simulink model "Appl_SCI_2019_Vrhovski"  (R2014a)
settings: Solver=ode45  StartTime=0.0  StopTime=1000  MaxStep=0.01  RelTol=1e-3
undefined symbols (not defined in the file): deg, H, kg, m, M, mm, N, rad, s, X, Y, Z
libraries: sm_lib x389, nesl_utility x69, simulink x7
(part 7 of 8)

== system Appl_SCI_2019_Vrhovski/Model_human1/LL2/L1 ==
  Mux : Mux  Inputs=3
  Pos X Converter : nesl_utility/PS-Simulink Converter  PhysicalDomain=network_engine_domain  SubClassName=ps_output  LeftPortType=input  RightPortType=output  PseudoPeriodic=off  Frequencies=[]  Unit=mm  AffineConversion=off
  Pos Y Converter : nesl_utility/PS-Simulink Converter  PhysicalDomain=network_engine_domain  SubClassName=ps_output  LeftPortType=input  RightPortType=output  PseudoPeriodic=off  Frequencies=[]  Unit=mm  AffineConversion=off
  Pos Z Converter2 : nesl_utility/PS-Simulink Converter  PhysicalDomain=network_engine_domain  SubClassName=ps_output  LeftPortType=input  RightPortType=output  PseudoPeriodic=off  Frequencies=[]  Unit=mm  AffineConversion=off
  Transform Sensor : sm_lib/Frames and Transforms/Transform Sensor  MeasurementFrame=World  SenseAngle=off  SenseAxis=off  SenseAngle1=off  SenseAngle2=off  SenseAngle3=off  SenseQ=off  SenseR=off  SenseOmegaX=off  SenseOmegaY=off  SenseOmegaZ=off  SenseOmega1=off  SenseOmega2=off  SenseOmega3=off  SenseQDot=off  SenseRDot=off  SenseAlphaX=off  SenseAlphaY=off  SenseAlphaZ=off  SenseAlpha1=off  SenseAlpha2=off  SenseAlpha3=off  SenseQDDot=off  SenseRDDot=off  SenseX=on  SenseY=on  SenseZ=on  SenseRad=on  SenseAzim=off  SenseDist=off  SenseInc=off  SenseXDot=off  SenseYDot=off  SenseZDot=off  SenseRadDot=off  SenseAzimDot=off  SenseDistDot=off  SenseIncDot=off  SenseXDDot=off  SenseYDDot=off  SenseZDDot=off  SenseRadDDot=off  SenseAzimDDot=off  SenseDistDDot=off  SenseIncDDot=off  BlockFunction=simmechanics.library.frames_transforms.transform_sensor
  base_coord_sys : PMIOPort  Port=1  Side=Left
  marker : PMIOPort  Port=2  Side=Left
  xyz : Outport
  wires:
  Pos Z Converter2/1 -> Mux/3
  Pos X Converter/1 -> Mux/1
  Pos Y Converter/1 -> Mux/2
  Mux/1 -> xyz/1
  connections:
  base_coord_sys/RConn1 -- Transform Sensor/LConn1
  marker/RConn1 -- Transform Sensor/RConn1
  Pos Z Converter2/LConn1 -- Transform Sensor/RConn4
  Pos X Converter/LConn1 -- Transform Sensor/RConn2
  Transform Sensor/RConn3 -- Pos Y Converter/LConn1

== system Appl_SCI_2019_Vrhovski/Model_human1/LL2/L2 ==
  Mux : Mux  Inputs=3
  Pos X Converter : nesl_utility/PS-Simulink Converter  PhysicalDomain=network_engine_domain  SubClassName=ps_output  LeftPortType=input  RightPortType=output  PseudoPeriodic=off  Frequencies=[]  Unit=mm  AffineConversion=off
  Pos Y Converter : nesl_utility/PS-Simulink Converter  PhysicalDomain=network_engine_domain  SubClassName=ps_output  LeftPortType=input  RightPortType=output  PseudoPeriodic=off  Frequencies=[]  Unit=mm  AffineConversion=off
  Pos Z Converter2 : nesl_utility/PS-Simulink Converter  PhysicalDomain=network_engine_domain  SubClassName=ps_output  LeftPortType=input  RightPortType=output  PseudoPeriodic=off  Frequencies=[]  Unit=mm  AffineConversion=off
  Transform Sensor : sm_lib/Frames and Transforms/Transform Sensor  MeasurementFrame=World  SenseAngle=off  SenseAxis=off  SenseAngle1=off  SenseAngle2=off  SenseAngle3=off  SenseQ=off  SenseR=off  SenseOmegaX=off  SenseOmegaY=off  SenseOmegaZ=off  SenseOmega1=off  SenseOmega2=off  SenseOmega3=off  SenseQDot=off  SenseRDot=off  SenseAlphaX=off  SenseAlphaY=off  SenseAlphaZ=off  SenseAlpha1=off  SenseAlpha2=off  SenseAlpha3=off  SenseQDDot=off  SenseRDDot=off  SenseX=on  SenseY=on  SenseZ=on  SenseRad=on  SenseAzim=off  SenseDist=off  SenseInc=off  SenseXDot=off  SenseYDot=off  SenseZDot=off  SenseRadDot=off  SenseAzimDot=off  SenseDistDot=off  SenseIncDot=off  SenseXDDot=off  SenseYDDot=off  SenseZDDot=off  SenseRadDDot=off  SenseAzimDDot=off  SenseDistDDot=off  SenseIncDDot=off  BlockFunction=simmechanics.library.frames_transforms.transform_sensor
  base_coord_sys : PMIOPort  Port=1  Side=Left
  marker : PMIOPort  Port=2  Side=Left
  xyz : Outport
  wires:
  Mux/1 -> xyz/1
  Pos Y Converter/1 -> Mux/2
  Pos X Converter/1 -> Mux/1
  Pos Z Converter2/1 -> Mux/3
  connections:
  Transform Sensor/RConn3 -- Pos Y Converter/LConn1
  Pos X Converter/LConn1 -- Transform Sensor/RConn2
  Pos Z Converter2/LConn1 -- Transform Sensor/RConn4
  marker/RConn1 -- Transform Sensor/RConn1
  base_coord_sys/RConn1 -- Transform Sensor/LConn1

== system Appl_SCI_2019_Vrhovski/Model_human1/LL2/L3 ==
  Mux : Mux  Inputs=3
  Pos X Converter : nesl_utility/PS-Simulink Converter  PhysicalDomain=network_engine_domain  SubClassName=ps_output  LeftPortType=input  RightPortType=output  PseudoPeriodic=off  Frequencies=[]  Unit=mm  AffineConversion=off
  Pos Y Converter : nesl_utility/PS-Simulink Converter  PhysicalDomain=network_engine_domain  SubClassName=ps_output  LeftPortType=input  RightPortType=output  PseudoPeriodic=off  Frequencies=[]  Unit=mm  AffineConversion=off
  Pos Z Converter2 : nesl_utility/PS-Simulink Converter  PhysicalDomain=network_engine_domain  SubClassName=ps_output  LeftPortType=input  RightPortType=output  PseudoPeriodic=off  Frequencies=[]  Unit=mm  AffineConversion=off
  Transform Sensor : sm_lib/Frames and Transforms/Transform Sensor  MeasurementFrame=World  SenseAngle=off  SenseAxis=off  SenseAngle1=off  SenseAngle2=off  SenseAngle3=off  SenseQ=off  SenseR=off  SenseOmegaX=off  SenseOmegaY=off  SenseOmegaZ=off  SenseOmega1=off  SenseOmega2=off  SenseOmega3=off  SenseQDot=off  SenseRDot=off  SenseAlphaX=off  SenseAlphaY=off  SenseAlphaZ=off  SenseAlpha1=off  SenseAlpha2=off  SenseAlpha3=off  SenseQDDot=off  SenseRDDot=off  SenseX=on  SenseY=on  SenseZ=on  SenseRad=on  SenseAzim=off  SenseDist=off  SenseInc=off  SenseXDot=off  SenseYDot=off  SenseZDot=off  SenseRadDot=off  SenseAzimDot=off  SenseDistDot=off  SenseIncDot=off  SenseXDDot=off  SenseYDDot=off  SenseZDDot=off  SenseRadDDot=off  SenseAzimDDot=off  SenseDistDDot=off  SenseIncDDot=off  BlockFunction=simmechanics.library.frames_transforms.transform_sensor
  base_coord_sys : PMIOPort  Port=1  Side=Left
  marker : PMIOPort  Port=2  Side=Left
  xyz : Outport
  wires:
  Pos Z Converter2/1 -> Mux/3
  Pos X Converter/1 -> Mux/1
  Pos Y Converter/1 -> Mux/2
  Mux/1 -> xyz/1
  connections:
  base_coord_sys/RConn1 -- Transform Sensor/LConn1
  marker/RConn1 -- Transform Sensor/RConn1
  Pos Z Converter2/LConn1 -- Transform Sensor/RConn4
  Pos X Converter/LConn1 -- Transform Sensor/RConn2
  Transform Sensor/RConn3 -- Pos Y Converter/LConn1

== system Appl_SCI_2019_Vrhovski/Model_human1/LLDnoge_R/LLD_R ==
  ReferenceFrame : sm_lib/Frames and Transforms/Reference Frame  BlockFunction=simmechanics.library.frames_transforms.reference_frame
  Solid : sm_lib/Body Elements/Solid  InertiaType=Custom  Mass=0  MassUnits=kg  CenterOfMass=[0 0 0]  CenterOfMassUnits=mm  MomentsOfInertia=[2897.1863857204326 1.8962829928219973 2897.1862300567827]  MomentsOfInertiaUnits=kg*mm^2  ProductsOfInertia=[0 0 -0.00027890183916846033]  ProductsOfInertiaUnits=kg*mm^2  DensityBased=on  Density=1000  DensityUnits=kg/(m^3)  GraphicType=FromGeometry  MarkerShape=Sphere  MarkerSize=10  MarkerSizeUnits=m  GraphicVisPropType=SimpleVisualProperties  GraphicDiffuseColor=[0.792156862745098 0.81960784313725488 0.93333333333333335]  GraphicSpecularColor=[0.5 0.5 0.5 1.0]  GraphicAmbientColor=[0.15 0.15 0.15 1.0]  GraphicEmissiveColor=[0.0 0.0 0.0 1.0]  GraphicShininess=75  GraphicOpacity=1  GeometryShape=Cylinder  RectangleSize=[1 1]  RectangleSizeUnits=m  BrickDimensions=[1 1 1]  BrickDimensionUnits=m  CylinderRadius=2.5  CylinderRadiusUnits=cm  CylinderLength=20  CylinderLengthUnits=cm  SphereRadius=5  SphereRadiusUnits=cm  EllipsoidRadii=[1 1 1]  EllipsoidRadiiUnits=m  ExtrusionCrossSection=[1 1; -1 1; -1 -1; 1 -1]  ExtrusionCrossSectionUnits=m  ExtrusionLength=1  ExtrusionLengthUnits=m  PolygonNumSides=3  PolygonOuterRadius=1  PolygonOuterRadiusUnits=m  ExtGeomFileType=STL  ExtGeomFileName=Pod_Default_sldprt.STL  ExtGeomFileUnits=mm  RevolutionCrossSection=[1 1; 1 -1; 2 -1; 2 1]  RevolutionCrossSectionUnits=m  RevolutionExtent=Full  RevolutionAngle=180  RevolutionAngleUnits=deg  BlockFunction=simmechanics.library.body_elements.solid
  Transform1 : sm_lib/Frames and Transforms/Rigid Transform  TranslationMethod=None  TranslationLengthUnit=mm  TranslationStandardAxis=-Z  TranslationStandardOffset=100  TranslationCartesianOffset=[1.3358203432289883e-12 650.00000000000045 -1.0913936421275139e-11]  TranslationROffset=0  TranslationROffsetUnits=m  TranslationZOffset=0  TranslationZOffsetUnits=m  TranslationThetaOffset=0  TranslationThetaOffsetUnits=deg  RotationMethod=None  RotationAngleUnits=rad  RotationStandardAxis=+Z  RotationAngle=0  RotationArbitraryAxis=[0 0 0]  FollAlignAxisA=+X  BaseAlignAxisA=+Y  FollAlignAxisB=+Y  BaseAlignAxisB=+Z  BlockFunction=simmechanics.library.frames_transforms.rigid_transform
  Transform2 : sm_lib/Frames and Transforms/Rigid Transform  TranslationMethod=None  TranslationLengthUnit=mm  TranslationStandardAxis=-Z  TranslationStandardOffset=100  TranslationCartesianOffset=[-2.2026824808563106e-13 549.99999999999943 3.4106051316484809e-13]  TranslationROffset=0  TranslationROffsetUnits=m  TranslationZOffset=0  TranslationZOffsetUnits=m  TranslationThetaOffset=0  TranslationThetaOffsetUnits=deg  RotationMethod=None  RotationAngleUnits=rad  RotationStandardAxis=+X  RotationAngle=pi/2  RotationArbitraryAxis=[0.57735026918962595 -0.57735026918962618 0.57735026918962518]  FollAlignAxisA=+X  BaseAlignAxisA=+Y  FollAlignAxisB=+Y  BaseAlignAxisB=+Z  BlockFunction=simmechanics.library.frames_transforms.rigid_transform
  F : PMIOPort  Port=1  Side=Right
  B : PMIOPort  Port=2  Side=Left
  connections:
  B/RConn1 -- Transform2/RConn1
  Transform1/RConn1 -- F/RConn1
  ReferenceFrame/RConn1 -- Solid/RConn1 -- Transform1/LConn1 -- Transform2/LConn1

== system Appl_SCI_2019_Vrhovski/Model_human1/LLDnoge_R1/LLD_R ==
  ReferenceFrame : sm_lib/Frames and Transforms/Reference Frame  BlockFunction=simmechanics.library.frames_transforms.reference_frame
  Solid : sm_lib/Body Elements/Solid  InertiaType=Custom  Mass=0  MassUnits=kg  CenterOfMass=[0 0 0]  CenterOfMassUnits=mm  MomentsOfInertia=[2897.1863857204326 1.8962829928219973 2897.1862300567827]  MomentsOfInertiaUnits=kg*mm^2  ProductsOfInertia=[0 0 -0.00027890183916846033]  ProductsOfInertiaUnits=kg*mm^2  DensityBased=on  Density=1000  DensityUnits=kg/(m^3)  GraphicType=FromGeometry  MarkerShape=Sphere  MarkerSize=10  MarkerSizeUnits=m  GraphicVisPropType=SimpleVisualProperties  GraphicDiffuseColor=[0.792156862745098 0.81960784313725488 0.93333333333333335]  GraphicSpecularColor=[0.5 0.5 0.5 1.0]  GraphicAmbientColor=[0.15 0.15 0.15 1.0]  GraphicEmissiveColor=[0.0 0.0 0.0 1.0]  GraphicShininess=75  GraphicOpacity=1  GeometryShape=Cylinder  RectangleSize=[1 1]  RectangleSizeUnits=m  BrickDimensions=[1 1 1]  BrickDimensionUnits=m  CylinderRadius=2.5  CylinderRadiusUnits=cm  CylinderLength=20  CylinderLengthUnits=cm  SphereRadius=5  SphereRadiusUnits=cm  EllipsoidRadii=[1 1 1]  EllipsoidRadiiUnits=m  ExtrusionCrossSection=[1 1; -1 1; -1 -1; 1 -1]  ExtrusionCrossSectionUnits=m  ExtrusionLength=1  ExtrusionLengthUnits=m  PolygonNumSides=3  PolygonOuterRadius=1  PolygonOuterRadiusUnits=m  ExtGeomFileType=STL  ExtGeomFileName=Pod_Default_sldprt.STL  ExtGeomFileUnits=mm  RevolutionCrossSection=[1 1; 1 -1; 2 -1; 2 1]  RevolutionCrossSectionUnits=m  RevolutionExtent=Full  RevolutionAngle=180  RevolutionAngleUnits=deg  BlockFunction=simmechanics.library.body_elements.solid
  Transform1 : sm_lib/Frames and Transforms/Rigid Transform  TranslationMethod=None  TranslationLengthUnit=mm  TranslationStandardAxis=-Z  TranslationStandardOffset=100  TranslationCartesianOffset=[1.3358203432289883e-12 650.00000000000045 -1.0913936421275139e-11]  TranslationROffset=0  TranslationROffsetUnits=m  TranslationZOffset=0  TranslationZOffsetUnits=m  TranslationThetaOffset=0  TranslationThetaOffsetUnits=deg  RotationMethod=None  RotationAngleUnits=rad  RotationStandardAxis=+Z  RotationAngle=0  RotationArbitraryAxis=[0 0 0]  FollAlignAxisA=+X  BaseAlignAxisA=+Y  FollAlignAxisB=+Y  BaseAlignAxisB=+Z  BlockFunction=simmechanics.library.frames_transforms.rigid_transform
  Transform2 : sm_lib/Frames and Transforms/Rigid Transform  TranslationMethod=None  TranslationLengthUnit=mm  TranslationStandardAxis=-Z  TranslationStandardOffset=100  TranslationCartesianOffset=[-2.2026824808563106e-13 549.99999999999943 3.4106051316484809e-13]  TranslationROffset=0  TranslationROffsetUnits=m  TranslationZOffset=0  TranslationZOffsetUnits=m  TranslationThetaOffset=0  TranslationThetaOffsetUnits=deg  RotationMethod=None  RotationAngleUnits=rad  RotationStandardAxis=+X  RotationAngle=pi/2  RotationArbitraryAxis=[0.57735026918962595 -0.57735026918962618 0.57735026918962518]  FollAlignAxisA=+X  BaseAlignAxisA=+Y  FollAlignAxisB=+Y  BaseAlignAxisB=+Z  BlockFunction=simmechanics.library.frames_transforms.rigid_transform
  F : PMIOPort  Port=1  Side=Right
  B : PMIOPort  Port=2  Side=Left
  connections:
  Transform2/LConn1 -- Transform1/LConn1 -- Solid/RConn1 -- ReferenceFrame/RConn1
  Transform1/RConn1 -- F/RConn1
  B/RConn1 -- Transform2/RConn1

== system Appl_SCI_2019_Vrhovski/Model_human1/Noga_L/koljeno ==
  ReferenceFrame : sm_lib/Frames and Transforms/Reference Frame  BlockFunction=simmechanics.library.frames_transforms.reference_frame
  Solid : sm_lib/Body Elements/Solid  InertiaType=Custom  Mass=0.0  MassUnits=kg  CenterOfMass=[0 0 0]  CenterOfMassUnits=mm  MomentsOfInertia=[2897.1863857204326 1.8962829928219973 2897.1862300567827]  MomentsOfInertiaUnits=kg*mm^2  ProductsOfInertia=[0 0 -0.00027890183916846033]  ProductsOfInertiaUnits=kg*mm^2  DensityBased=on  Density=1000  DensityUnits=kg/(m^3)  GraphicType=FromGeometry  MarkerShape=Sphere  MarkerSize=10  MarkerSizeUnits=m  GraphicVisPropType=SimpleVisualProperties  GraphicDiffuseColor=[0.792156862745098 0.81960784313725488 0.93333333333333335]  GraphicSpecularColor=[0.5 0.5 0.5 1.0]  GraphicAmbientColor=[0.15 0.15 0.15 1.0]  GraphicEmissiveColor=[0.0 0.0 0.0 1.0]  GraphicShininess=75  GraphicOpacity=1  GeometryShape=Sphere  RectangleSize=[1 1]  RectangleSizeUnits=m  BrickDimensions=[1 1 1]  BrickDimensionUnits=m  CylinderRadius=1  CylinderRadiusUnits=m  CylinderLength=1  CylinderLengthUnits=m  SphereRadius=3  SphereRadiusUnits=cm  EllipsoidRadii=[1 1 1]  EllipsoidRadiiUnits=m  ExtrusionCrossSection=[1 1; -1 1; -1 -1; 1 -1]  ExtrusionCrossSectionUnits=m  ExtrusionLength=1  ExtrusionLengthUnits=m  PolygonNumSides=3  PolygonOuterRadius=1  PolygonOuterRadiusUnits=m  ExtGeomFileType=STL  ExtGeomFileName=Pod_Default_sldprt.STL  ExtGeomFileUnits=mm  RevolutionCrossSection=[1 1; 1 -1; 2 -1; 2 1]  RevolutionCrossSectionUnits=m  RevolutionExtent=Full  RevolutionAngle=180  RevolutionAngleUnits=deg  BlockFunction=simmechanics.library.body_elements.solid
  Transform : sm_lib/Frames and Transforms/Rigid Transform  TranslationMethod=None  TranslationLengthUnit=mm  TranslationStandardAxis=+Z  TranslationStandardOffset=0  TranslationCartesianOffset=[-2.2026824808563106e-13 549.99999999999943 3.4106051316484809e-13]  TranslationROffset=0  TranslationROffsetUnits=m  TranslationZOffset=0  TranslationZOffsetUnits=m  TranslationThetaOffset=0  TranslationThetaOffsetUnits=deg  RotationMethod=None  RotationAngleUnits=rad  RotationStandardAxis=+Z  RotationAngle=2.0943951023931962  RotationArbitraryAxis=[0.57735026918962595 -0.57735026918962618 0.57735026918962518]  FollAlignAxisA=+X  BaseAlignAxisA=+Y  FollAlignAxisB=+Y  BaseAlignAxisB=+Z  BlockFunction=simmechanics.library.frames_transforms.rigid_transform
  Transform1 : sm_lib/Frames and Transforms/Rigid Transform  TranslationMethod=None  TranslationLengthUnit=mm  TranslationStandardAxis=+Z  TranslationStandardOffset=0  TranslationCartesianOffset=[1.3358203432289883e-12 0 -1.0913936421275139e-11]  TranslationROffset=0  TranslationROffsetUnits=m  TranslationZOffset=0  TranslationZOffsetUnits=m  TranslationThetaOffset=0  TranslationThetaOffsetUnits=deg  RotationMethod=None  RotationAngleUnits=rad  RotationStandardAxis=+X  RotationAngle=pi/2  RotationArbitraryAxis=[0 0 0]  FollAlignAxisA=+X  BaseAlignAxisA=+Y  FollAlignAxisB=+Y  BaseAlignAxisB=+Z  BlockFunction=simmechanics.library.frames_transforms.rigid_transform
  F : PMIOPort  Port=1  Side=Right
  B : PMIOPort  Port=2  Side=Left
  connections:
  Transform1/RConn1 -- F/RConn1
  Transform/RConn1 -- B/RConn1
  Solid/RConn1 -- ReferenceFrame/RConn1 -- Transform1/LConn1 -- Transform/LConn1

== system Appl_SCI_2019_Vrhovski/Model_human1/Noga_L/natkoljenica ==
  ReferenceFrame : sm_lib/Frames and Transforms/Reference Frame  BlockFunction=simmechanics.library.frames_transforms.reference_frame
  Solid : sm_lib/Body Elements/Solid  InertiaType=Custom  Mass=0.1416*M  MassUnits=kg  CenterOfMass=[0 0 0]  CenterOfMassUnits=mm  MomentsOfInertia=[2897.1863857204326 1.8962829928219973 2897.1862300567827]  MomentsOfInertiaUnits=kg*mm^2  ProductsOfInertia=[0 0 -0.00027890183916846033]  ProductsOfInertiaUnits=kg*mm^2  DensityBased=on  Density=1000  DensityUnits=kg/(m^3)  GraphicType=FromGeometry  MarkerShape=Sphere  MarkerSize=10  MarkerSizeUnits=m  GraphicVisPropType=SimpleVisualProperties  GraphicDiffuseColor=[0.792156862745098 0.81960784313725488 0.93333333333333335]  GraphicSpecularColor=[0.5 0.5 0.5 1.0]  GraphicAmbientColor=[0.15 0.15 0.15 1.0]  GraphicEmissiveColor=[0.0 0.0 0.0 1.0]  GraphicShininess=75  GraphicOpacity=1  GeometryShape=Ellipsoid  RectangleSize=[1 1]  RectangleSizeUnits=m  BrickDimensions=[1 1 1]  BrickDimensionUnits=m  CylinderRadius=2.5  CylinderRadiusUnits=cm  CylinderLength=50  CylinderLengthUnits=cm  SphereRadius=5  SphereRadiusUnits=cm  EllipsoidRadii=[60 60 0.195*H*5]  EllipsoidRadiiUnits=mm  ExtrusionCrossSection=[1 1; -1 1; -1 -1; 1 -1]  ExtrusionCrossSectionUnits=m  ExtrusionLength=1  ExtrusionLengthUnits=m  PolygonNumSides=3  PolygonOuterRadius=1  PolygonOuterRadiusUnits=m  ExtGeomFileType=STL  ExtGeomFileName=Pod_Default_sldprt.STL  ExtGeomFileUnits=mm  RevolutionCrossSection=[1 1; 1 -1; 2 -1; 2 1]  RevolutionCrossSectionUnits=m  RevolutionExtent=Full  RevolutionAngle=180  RevolutionAngleUnits=deg  BlockFunction=simmechanics.library.body_elements.solid
  Transform1 : sm_lib/Frames and Transforms/Rigid Transform  TranslationMethod=StandardAxis  TranslationLengthUnit=mm  TranslationStandardAxis=+Z  TranslationStandardOffset=0.195*H*5  TranslationCartesianOffset=[1.3358203432289883e-12 650.00000000000045 -1.0913936421275139e-11]  TranslationROffset=0  TranslationROffsetUnits=m  TranslationZOffset=0  TranslationZOffsetUnits=m  TranslationThetaOffset=0  TranslationThetaOffsetUnits=deg  RotationMethod=None  RotationAngleUnits=rad  RotationStandardAxis=+Z  RotationAngle=0  RotationArbitraryAxis=[0 0 0]  FollAlignAxisA=+X  BaseAlignAxisA=+Y  FollAlignAxisB=+Y  BaseAlignAxisB=+Z  BlockFunction=simmechanics.library.frames_transforms.rigid_transform
  Transform2 : sm_lib/Frames and Transforms/Rigid Transform  TranslationMethod=StandardAxis  TranslationLengthUnit=mm  TranslationStandardAxis=-Z  TranslationStandardOffset=0.195*H*5  TranslationCartesianOffset=[-2.2026824808563106e-13 549.99999999999943 3.4106051316484809e-13]  TranslationROffset=0  TranslationROffsetUnits=m  TranslationZOffset=0  TranslationZOffsetUnits=m  TranslationThetaOffset=0  TranslationThetaOffsetUnits=deg  RotationMethod=None  RotationAngleUnits=rad  RotationStandardAxis=+X  RotationAngle=pi/2  RotationArbitraryAxis=[0.57735026918962595 -0.57735026918962618 0.57735026918962518]  FollAlignAxisA=+X  BaseAlignAxisA=+Y  FollAlignAxisB=+Y  BaseAlignAxisB=+Z  BlockFunction=simmechanics.library.frames_transforms.rigid_transform
  F : PMIOPort  Port=1  Side=Right
  B : PMIOPort  Port=2  Side=Left
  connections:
  Transform2/LConn1 -- Transform1/LConn1 -- Solid/RConn1 -- ReferenceFrame/RConn1
  Transform1/RConn1 -- F/RConn1
  B/RConn1 -- Transform2/RConn1

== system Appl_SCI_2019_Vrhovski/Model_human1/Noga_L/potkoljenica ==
  ReferenceFrame : sm_lib/Frames and Transforms/Reference Frame  BlockFunction=simmechanics.library.frames_transforms.reference_frame
  Solid : sm_lib/Body Elements/Solid  InertiaType=Custom  Mass=0.0433*M  MassUnits=kg  CenterOfMass=[0 0 0]  CenterOfMassUnits=mm  MomentsOfInertia=[2897.1863857204326 1.8962829928219973 2897.1862300567827]  MomentsOfInertiaUnits=kg*mm^2  ProductsOfInertia=[0 0 -0.00027890183916846033]  ProductsOfInertiaUnits=kg*mm^2  DensityBased=on  Density=1000  DensityUnits=kg/(m^3)  GraphicType=FromGeometry  MarkerShape=Sphere  MarkerSize=10  MarkerSizeUnits=m  GraphicVisPropType=SimpleVisualProperties  GraphicDiffuseColor=[0.792156862745098 0.81960784313725488 0.93333333333333335]  GraphicSpecularColor=[0.5 0.5 0.5 1.0]  GraphicAmbientColor=[0.15 0.15 0.15 1.0]  GraphicEmissiveColor=[0.0 0.0 0.0 1.0]  GraphicShininess=75  GraphicOpacity=1  GeometryShape=Ellipsoid  RectangleSize=[1 1]  RectangleSizeUnits=m  BrickDimensions=[1 1 1]  BrickDimensionUnits=m  CylinderRadius=2.5  CylinderRadiusUnits=cm  CylinderLength=50  CylinderLengthUnits=cm  SphereRadius=5  SphereRadiusUnits=cm  EllipsoidRadii=[50 50 0.246*H*5]  EllipsoidRadiiUnits=mm  ExtrusionCrossSection=[1 1; -1 1; -1 -1; 1 -1]  ExtrusionCrossSectionUnits=m  ExtrusionLength=1  ExtrusionLengthUnits=m  PolygonNumSides=3  PolygonOuterRadius=1  PolygonOuterRadiusUnits=m  ExtGeomFileType=STL  ExtGeomFileName=Pod_Default_sldprt.STL  ExtGeomFileUnits=mm  RevolutionCrossSection=[1 1; 1 -1; 2 -1; 2 1]  RevolutionCrossSectionUnits=m  RevolutionExtent=Full  RevolutionAngle=180  RevolutionAngleUnits=deg  BlockFunction=simmechanics.library.body_elements.solid
  Transform1 : sm_lib/Frames and Transforms/Rigid Transform  TranslationMethod=StandardAxis  TranslationLengthUnit=mm  TranslationStandardAxis=+Z  TranslationStandardOffset=0.246*H*5  TranslationCartesianOffset=[1.3358203432289883e-12 650.00000000000045 -1.0913936421275139e-11]  TranslationROffset=0  TranslationROffsetUnits=m  TranslationZOffset=0  TranslationZOffsetUnits=m  TranslationThetaOffset=0  TranslationThetaOffsetUnits=deg  RotationMethod=None  RotationAngleUnits=rad  RotationStandardAxis=+Z  RotationAngle=0  RotationArbitraryAxis=[0 0 0]  FollAlignAxisA=+X  BaseAlignAxisA=+Y  FollAlignAxisB=+Y  BaseAlignAxisB=+Z  BlockFunction=simmechanics.library.frames_transforms.rigid_transform
  Transform2 : sm_lib/Frames and Transforms/Rigid Transform  TranslationMethod=StandardAxis  TranslationLengthUnit=mm  TranslationStandardAxis=-Z  TranslationStandardOffset=0.246*H*5  TranslationCartesianOffset=[-2.2026824808563106e-13 549.99999999999943 3.4106051316484809e-13]  TranslationROffset=0  TranslationROffsetUnits=m  TranslationZOffset=0  TranslationZOffsetUnits=m  TranslationThetaOffset=0  TranslationThetaOffsetUnits=deg  RotationMethod=None  RotationAngleUnits=rad  RotationStandardAxis=+X  RotationAngle=pi/2  RotationArbitraryAxis=[0.57735026918962595 -0.57735026918962618 0.57735026918962518]  FollAlignAxisA=+X  BaseAlignAxisA=+Y  FollAlignAxisB=+Y  BaseAlignAxisB=+Z  BlockFunction=simmechanics.library.frames_transforms.rigid_transform
  F : PMIOPort  Port=1  Side=Right
  B : PMIOPort  Port=2  Side=Left
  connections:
  B/RConn1 -- Transform2/RConn1
  Transform1/RConn1 -- F/RConn1
  Transform2/LConn1 -- Transform1/LConn1 -- ReferenceFrame/RConn1 -- Solid/RConn1

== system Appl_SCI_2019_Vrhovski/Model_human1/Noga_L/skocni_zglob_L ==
  ReferenceFrame : sm_lib/Frames and Transforms/Reference Frame  BlockFunction=simmechanics.library.frames_transforms.reference_frame
  Solid : sm_lib/Body Elements/Solid  InertiaType=Custom  Mass=0.0137*M  MassUnits=kg  CenterOfMass=[0 0 0]  CenterOfMassUnits=mm  MomentsOfInertia=[2897.1863857204326 1.8962829928219973 2897.1862300567827]  MomentsOfInertiaUnits=kg*mm^2  ProductsOfInertia=[0 0 -0.00027890183916846033]  ProductsOfInertiaUnits=kg*mm^2  DensityBased=on  Density=1000  DensityUnits=kg/(m^3)  GraphicType=FromGeometry  MarkerShape=Sphere  MarkerSize=10  MarkerSizeUnits=m  GraphicVisPropType=SimpleVisualProperties  GraphicDiffuseColor=[0.792156862745098 0.81960784313725488 0.93333333333333335]  GraphicSpecularColor=[0.5 0.5 0.5 1.0]  GraphicAmbientColor=[0.15 0.15 0.15 1.0]  GraphicEmissiveColor=[0.0 0.0 0.0 1.0]  GraphicShininess=75  GraphicOpacity=1  GeometryShape=Sphere  RectangleSize=[1 1]  RectangleSizeUnits=m  BrickDimensions=[1 1 1]  BrickDimensionUnits=m  CylinderRadius=1  CylinderRadiusUnits=m  CylinderLength=1  CylinderLengthUnits=m  SphereRadius=0.039*H/2  SphereRadiusUnits=cm  EllipsoidRadii=[1 1 1]  EllipsoidRadiiUnits=m  ExtrusionCrossSection=[1 1; -1 1; -1 -1; 1 -1]  ExtrusionCrossSectionUnits=m  ExtrusionLength=1  ExtrusionLengthUnits=m  PolygonNumSides=3  PolygonOuterRadius=1  PolygonOuterRadiusUnits=m  ExtGeomFileType=STL  ExtGeomFileName=Pod_Default_sldprt.STL  ExtGeomFileUnits=mm  RevolutionCrossSection=[1 1; 1 -1; 2 -1; 2 1]  RevolutionCrossSectionUnits=m  RevolutionExtent=Full  RevolutionAngle=180  RevolutionAngleUnits=deg  BlockFunction=simmechanics.library.body_elements.solid
  Transform : sm_lib/Frames and Transforms/Rigid Transform  TranslationMethod=None  TranslationLengthUnit=mm  TranslationStandardAxis=+Z  TranslationStandardOffset=0  TranslationCartesianOffset=[-2.2026824808563106e-13 549.99999999999943 3.4106051316484809e-13]  TranslationROffset=0  TranslationROffsetUnits=m  TranslationZOffset=0  TranslationZOffsetUnits=m  TranslationThetaOffset=0  TranslationThetaOffsetUnits=deg  RotationMethod=None  RotationAngleUnits=rad  RotationStandardAxis=+Z  RotationAngle=2.0943951023931962  RotationArbitraryAxis=[0.57735026918962595 -0.57735026918962618 0.57735026918962518]  FollAlignAxisA=+X  BaseAlignAxisA=+Y  FollAlignAxisB=+Y  BaseAlignAxisB=+Z  BlockFunction=simmechanics.library.frames_transforms.rigid_transform
  Transform1 : sm_lib/Frames and Transforms/Rigid Transform  TranslationMethod=None  TranslationLengthUnit=mm  TranslationStandardAxis=+Z  TranslationStandardOffset=0  TranslationCartesianOffset=[1.3358203432289883e-12 0 -1.0913936421275139e-11]  TranslationROffset=0  TranslationROffsetUnits=m  TranslationZOffset=0  TranslationZOffsetUnits=m  TranslationThetaOffset=0  TranslationThetaOffsetUnits=deg  RotationMethod=None  RotationAngleUnits=rad  RotationStandardAxis=+X  RotationAngle=pi/2  RotationArbitraryAxis=[0 0 0]  FollAlignAxisA=+X  BaseAlignAxisA=+Y  FollAlignAxisB=+Y  BaseAlignAxisB=+Z  BlockFunction=simmechanics.library.frames_transforms.rigid_transform
  F : PMIOPort  Port=1  Side=Right
  B : PMIOPort  Port=2  Side=Left
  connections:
  Transform1/RConn1 -- F/RConn1
  Transform/RConn1 -- B/RConn1
  Solid/RConn1 -- ReferenceFrame/RConn1 -- Transform1/LConn1 -- Transform/LConn1

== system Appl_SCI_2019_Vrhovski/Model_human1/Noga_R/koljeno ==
  ReferenceFrame : sm_lib/Frames and Transforms/Reference Frame  BlockFunction=simmechanics.library.frames_transforms.reference_frame
  Solid : sm_lib/Body Elements/Solid  InertiaType=Custom  Mass=0.0  MassUnits=kg  CenterOfMass=[0 0 0]  CenterOfMassUnits=mm  MomentsOfInertia=[2897.1863857204326 1.8962829928219973 2897.1862300567827]  MomentsOfInertiaUnits=kg*mm^2  ProductsOfInertia=[0 0 -0.00027890183916846033]  ProductsOfInertiaUnits=kg*mm^2  DensityBased=on  Density=1000  DensityUnits=kg/(m^3)  GraphicType=FromGeometry  MarkerShape=Sphere  MarkerSize=10  MarkerSizeUnits=m  GraphicVisPropType=SimpleVisualProperties  GraphicDiffuseColor=[0.792156862745098 0.81960784313725488 0.93333333333333335]  GraphicSpecularColor=[0.5 0.5 0.5 1.0]  GraphicAmbientColor=[0.15 0.15 0.15 1.0]  GraphicEmissiveColor=[0.0 0.0 0.0 1.0]  GraphicShininess=75  GraphicOpacity=1  GeometryShape=Sphere  RectangleSize=[1 1]  RectangleSizeUnits=m  BrickDimensions=[1 1 1]  BrickDimensionUnits=m  CylinderRadius=1  CylinderRadiusUnits=m  CylinderLength=1  CylinderLengthUnits=m  SphereRadius=3  SphereRadiusUnits=cm  EllipsoidRadii=[1 1 1]  EllipsoidRadiiUnits=m  ExtrusionCrossSection=[1 1; -1 1; -1 -1; 1 -1]  ExtrusionCrossSectionUnits=m  ExtrusionLength=1  ExtrusionLengthUnits=m  PolygonNumSides=3  PolygonOuterRadius=1  PolygonOuterRadiusUnits=m  ExtGeomFileType=STL  ExtGeomFileName=Pod_Default_sldprt.STL  ExtGeomFileUnits=mm  RevolutionCrossSection=[1 1; 1 -1; 2 -1; 2 1]  RevolutionCrossSectionUnits=m  RevolutionExtent=Full  RevolutionAngle=180  RevolutionAngleUnits=deg  BlockFunction=simmechanics.library.body_elements.solid
  Transform : sm_lib/Frames and Transforms/Rigid Transform  TranslationMethod=None  TranslationLengthUnit=mm  TranslationStandardAxis=+Z  TranslationStandardOffset=0  TranslationCartesianOffset=[-2.2026824808563106e-13 549.99999999999943 3.4106051316484809e-13]  TranslationROffset=0  TranslationROffsetUnits=m  TranslationZOffset=0  TranslationZOffsetUnits=m  TranslationThetaOffset=0  TranslationThetaOffsetUnits=deg  RotationMethod=None  RotationAngleUnits=rad  RotationStandardAxis=+Z  RotationAngle=2.0943951023931962  RotationArbitraryAxis=[0.57735026918962595 -0.57735026918962618 0.57735026918962518]  FollAlignAxisA=+X  BaseAlignAxisA=+Y  FollAlignAxisB=+Y  BaseAlignAxisB=+Z  BlockFunction=simmechanics.library.frames_transforms.rigid_transform
  Transform1 : sm_lib/Frames and Transforms/Rigid Transform  TranslationMethod=None  TranslationLengthUnit=mm  TranslationStandardAxis=+Z  TranslationStandardOffset=0  TranslationCartesianOffset=[1.3358203432289883e-12 0 -1.0913936421275139e-11]  TranslationROffset=0  TranslationROffsetUnits=m  TranslationZOffset=0  TranslationZOffsetUnits=m  TranslationThetaOffset=0  TranslationThetaOffsetUnits=deg  RotationMethod=None  RotationAngleUnits=rad  RotationStandardAxis=+X  RotationAngle=pi/2  RotationArbitraryAxis=[0 0 0]  FollAlignAxisA=+X  BaseAlignAxisA=+Y  FollAlignAxisB=+Y  BaseAlignAxisB=+Z  BlockFunction=simmechanics.library.frames_transforms.rigid_transform
  F : PMIOPort  Port=1  Side=Right
  B : PMIOPort  Port=2  Side=Left
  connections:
  Transform1/RConn1 -- F/RConn1
  Transform/RConn1 -- B/RConn1
  Solid/RConn1 -- ReferenceFrame/RConn1 -- Transform1/LConn1 -- Transform/LConn1

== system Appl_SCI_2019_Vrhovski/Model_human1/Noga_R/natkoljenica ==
  ReferenceFrame : sm_lib/Frames and Transforms/Reference Frame  BlockFunction=simmechanics.library.frames_transforms.reference_frame
  Solid : sm_lib/Body Elements/Solid  InertiaType=Custom  Mass=0.1416*M  MassUnits=kg  CenterOfMass=[0 0 0]  CenterOfMassUnits=mm  MomentsOfInertia=[2897.1863857204326 1.8962829928219973 2897.1862300567827]  MomentsOfInertiaUnits=kg*mm^2  ProductsOfInertia=[0 0 -0.00027890183916846033]  ProductsOfInertiaUnits=kg*mm^2  DensityBased=on  Density=1000  DensityUnits=kg/(m^3)  GraphicType=FromGeometry  MarkerShape=Sphere  MarkerSize=10  MarkerSizeUnits=m  GraphicVisPropType=SimpleVisualProperties  GraphicDiffuseColor=[0.792156862745098 0.81960784313725488 0.93333333333333335]  GraphicSpecularColor=[0.5 0.5 0.5 1.0]  GraphicAmbientColor=[0.15 0.15 0.15 1.0]  GraphicEmissiveColor=[0.0 0.0 0.0 1.0]  GraphicShininess=75  GraphicOpacity=1  GeometryShape=Ellipsoid  RectangleSize=[1 1]  RectangleSizeUnits=m  BrickDimensions=[1 1 1]  BrickDimensionUnits=m  CylinderRadius=2.5  CylinderRadiusUnits=cm  CylinderLength=50  CylinderLengthUnits=cm  SphereRadius=5  SphereRadiusUnits=cm  EllipsoidRadii=[60 60 0.195*H*5]  EllipsoidRadiiUnits=mm  ExtrusionCrossSection=[1 1; -1 1; -1 -1; 1 -1]  ExtrusionCrossSectionUnits=m  ExtrusionLength=1  ExtrusionLengthUnits=m  PolygonNumSides=3  PolygonOuterRadius=1  PolygonOuterRadiusUnits=m  ExtGeomFileType=STL  ExtGeomFileName=Pod_Default_sldprt.STL  ExtGeomFileUnits=mm  RevolutionCrossSection=[1 1; 1 -1; 2 -1; 2 1]  RevolutionCrossSectionUnits=m  RevolutionExtent=Full  RevolutionAngle=180  RevolutionAngleUnits=deg  BlockFunction=simmechanics.library.body_elements.solid
  Transform1 : sm_lib/Frames and Transforms/Rigid Transform  TranslationMethod=StandardAxis  TranslationLengthUnit=mm  TranslationStandardAxis=+Z  TranslationStandardOffset=0.195*H*5  TranslationCartesianOffset=[1.3358203432289883e-12 650.00000000000045 -1.0913936421275139e-11]  TranslationROffset=0  TranslationROffsetUnits=m  TranslationZOffset=0  TranslationZOffsetUnits=m  TranslationThetaOffset=0  TranslationThetaOffsetUnits=deg  RotationMethod=None  RotationAngleUnits=rad  RotationStandardAxis=+Z  RotationAngle=0  RotationArbitraryAxis=[0 0 0]  FollAlignAxisA=+X  BaseAlignAxisA=+Y  FollAlignAxisB=+Y  BaseAlignAxisB=+Z  BlockFunction=simmechanics.library.frames_transforms.rigid_transform
  Transform2 : sm_lib/Frames and Transforms/Rigid Transform  TranslationMethod=StandardAxis  TranslationLengthUnit=mm  TranslationStandardAxis=-Z  TranslationStandardOffset=0.195*H*5  TranslationCartesianOffset=[-2.2026824808563106e-13 549.99999999999943 3.4106051316484809e-13]  TranslationROffset=0  TranslationROffsetUnits=m  TranslationZOffset=0  TranslationZOffsetUnits=m  TranslationThetaOffset=0  TranslationThetaOffsetUnits=deg  RotationMethod=None  RotationAngleUnits=rad  RotationStandardAxis=+X  RotationAngle=pi/2  RotationArbitraryAxis=[0.57735026918962595 -0.57735026918962618 0.57735026918962518]  FollAlignAxisA=+X  BaseAlignAxisA=+Y  FollAlignAxisB=+Y  BaseAlignAxisB=+Z  BlockFunction=simmechanics.library.frames_transforms.rigid_transform
  F : PMIOPort  Port=1  Side=Right
  B : PMIOPort  Port=2  Side=Left
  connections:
  Transform2/LConn1 -- Transform1/LConn1 -- Solid/RConn1 -- ReferenceFrame/RConn1
  Transform1/RConn1 -- F/RConn1
  B/RConn1 -- Transform2/RConn1

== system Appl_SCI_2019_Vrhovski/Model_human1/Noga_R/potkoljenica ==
  ReferenceFrame : sm_lib/Frames and Transforms/Reference Frame  BlockFunction=simmechanics.library.frames_transforms.reference_frame
  Solid : sm_lib/Body Elements/Solid  InertiaType=Custom  Mass=0.0433*M  MassUnits=kg  CenterOfMass=[0 0 0]  CenterOfMassUnits=mm  MomentsOfInertia=[2897.1863857204326 1.8962829928219973 2897.1862300567827]  MomentsOfInertiaUnits=kg*mm^2  ProductsOfInertia=[0 0 -0.00027890183916846033]  ProductsOfInertiaUnits=kg*mm^2  DensityBased=on  Density=1000  DensityUnits=kg/(m^3)  GraphicType=FromGeometry  MarkerShape=Sphere  MarkerSize=10  MarkerSizeUnits=m  GraphicVisPropType=SimpleVisualProperties  GraphicDiffuseColor=[0.792156862745098 0.81960784313725488 0.93333333333333335]  GraphicSpecularColor=[0.5 0.5 0.5 1.0]  GraphicAmbientColor=[0.15 0.15 0.15 1.0]  GraphicEmissiveColor=[0.0 0.0 0.0 1.0]  GraphicShininess=75  GraphicOpacity=1  GeometryShape=Ellipsoid  RectangleSize=[1 1]  RectangleSizeUnits=m  BrickDimensions=[1 1 1]  BrickDimensionUnits=m  CylinderRadius=2.5  CylinderRadiusUnits=cm  CylinderLength=50  CylinderLengthUnits=cm  SphereRadius=5  SphereRadiusUnits=cm  EllipsoidRadii=[50 50 0.246*H*5]  EllipsoidRadiiUnits=mm  ExtrusionCrossSection=[1 1; -1 1; -1 -1; 1 -1]  ExtrusionCrossSectionUnits=m  ExtrusionLength=1  ExtrusionLengthUnits=m  PolygonNumSides=3  PolygonOuterRadius=1  PolygonOuterRadiusUnits=m  ExtGeomFileType=STL  ExtGeomFileName=Pod_Default_sldprt.STL  ExtGeomFileUnits=mm  RevolutionCrossSection=[1 1; 1 -1; 2 -1; 2 1]  RevolutionCrossSectionUnits=m  RevolutionExtent=Full  RevolutionAngle=180  RevolutionAngleUnits=deg  BlockFunction=simmechanics.library.body_elements.solid
  Transform1 : sm_lib/Frames and Transforms/Rigid Transform  TranslationMethod=StandardAxis  TranslationLengthUnit=mm  TranslationStandardAxis=+Z  TranslationStandardOffset=0.246*H*5  TranslationCartesianOffset=[1.3358203432289883e-12 650.00000000000045 -1.0913936421275139e-11]  TranslationROffset=0  TranslationROffsetUnits=m  TranslationZOffset=0  TranslationZOffsetUnits=m  TranslationThetaOffset=0  TranslationThetaOffsetUnits=deg  RotationMethod=None  RotationAngleUnits=rad  RotationStandardAxis=+Z  RotationAngle=0  RotationArbitraryAxis=[0 0 0]  FollAlignAxisA=+X  BaseAlignAxisA=+Y  FollAlignAxisB=+Y  BaseAlignAxisB=+Z  BlockFunction=simmechanics.library.frames_transforms.rigid_transform
  Transform2 : sm_lib/Frames and Transforms/Rigid Transform  TranslationMethod=StandardAxis  TranslationLengthUnit=mm  TranslationStandardAxis=-Z  TranslationStandardOffset=0.246*H*5  TranslationCartesianOffset=[-2.2026824808563106e-13 549.99999999999943 3.4106051316484809e-13]  TranslationROffset=0  TranslationROffsetUnits=m  TranslationZOffset=0  TranslationZOffsetUnits=m  TranslationThetaOffset=0  TranslationThetaOffsetUnits=deg  RotationMethod=None  RotationAngleUnits=rad  RotationStandardAxis=+X  RotationAngle=pi/2  RotationArbitraryAxis=[0.57735026918962595 -0.57735026918962618 0.57735026918962518]  FollAlignAxisA=+X  BaseAlignAxisA=+Y  FollAlignAxisB=+Y  BaseAlignAxisB=+Z  BlockFunction=simmechanics.library.frames_transforms.rigid_transform
  F : PMIOPort  Port=1  Side=Right
  B : PMIOPort  Port=2  Side=Left
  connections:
  B/RConn1 -- Transform2/RConn1
  Transform1/RConn1 -- F/RConn1
  Transform2/LConn1 -- Transform1/LConn1 -- ReferenceFrame/RConn1 -- Solid/RConn1

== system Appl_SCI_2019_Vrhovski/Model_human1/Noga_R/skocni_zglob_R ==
  ReferenceFrame : sm_lib/Frames and Transforms/Reference Frame  BlockFunction=simmechanics.library.frames_transforms.reference_frame
  Solid : sm_lib/Body Elements/Solid  InertiaType=Custom  Mass=0.0137*M  MassUnits=kg  CenterOfMass=[0 0 0]  CenterOfMassUnits=mm  MomentsOfInertia=[2897.1863857204326 1.8962829928219973 2897.1862300567827]  MomentsOfInertiaUnits=kg*mm^2  ProductsOfInertia=[0 0 -0.00027890183916846033]  ProductsOfInertiaUnits=kg*mm^2  DensityBased=on  Density=1000  DensityUnits=kg/(m^3)  GraphicType=FromGeometry  MarkerShape=Sphere  MarkerSize=10  MarkerSizeUnits=m  GraphicVisPropType=SimpleVisualProperties  GraphicDiffuseColor=[0.792156862745098 0.81960784313725488 0.93333333333333335]  GraphicSpecularColor=[0.5 0.5 0.5 1.0]  GraphicAmbientColor=[0.15 0.15 0.15 1.0]  GraphicEmissiveColor=[0.0 0.0 0.0 1.0]  GraphicShininess=75  GraphicOpacity=1  GeometryShape=Sphere  RectangleSize=[1 1]  RectangleSizeUnits=m  BrickDimensions=[1 1 1]  BrickDimensionUnits=m  CylinderRadius=1  CylinderRadiusUnits=m  CylinderLength=1  CylinderLengthUnits=m  SphereRadius=0.039*H/2  SphereRadiusUnits=cm  EllipsoidRadii=[1 1 1]  EllipsoidRadiiUnits=m  ExtrusionCrossSection=[1 1; -1 1; -1 -1; 1 -1]  ExtrusionCrossSectionUnits=m  ExtrusionLength=1  ExtrusionLengthUnits=m  PolygonNumSides=3  PolygonOuterRadius=1  PolygonOuterRadiusUnits=m  ExtGeomFileType=STL  ExtGeomFileName=Pod_Default_sldprt.STL  ExtGeomFileUnits=mm  RevolutionCrossSection=[1 1; 1 -1; 2 -1; 2 1]  RevolutionCrossSectionUnits=m  RevolutionExtent=Full  RevolutionAngle=180  RevolutionAngleUnits=deg  BlockFunction=simmechanics.library.body_elements.solid
  Transform : sm_lib/Frames and Transforms/Rigid Transform  TranslationMethod=None  TranslationLengthUnit=mm  TranslationStandardAxis=+Z  TranslationStandardOffset=0  TranslationCartesianOffset=[-2.2026824808563106e-13 549.99999999999943 3.4106051316484809e-13]  TranslationROffset=0  TranslationROffsetUnits=m  TranslationZOffset=0  TranslationZOffsetUnits=m  TranslationThetaOffset=0  TranslationThetaOffsetUnits=deg  RotationMethod=None  RotationAngleUnits=rad  RotationStandardAxis=+Z  RotationAngle=2.0943951023931962  RotationArbitraryAxis=[0.57735026918962595 -0.57735026918962618 0.57735026918962518]  FollAlignAxisA=+X  BaseAlignAxisA=+Y  FollAlignAxisB=+Y  BaseAlignAxisB=+Z  BlockFunction=simmechanics.library.frames_transforms.rigid_transform
  Transform1 : sm_lib/Frames and Transforms/Rigid Transform  TranslationMethod=None  TranslationLengthUnit=mm  TranslationStandardAxis=+Z  TranslationStandardOffset=0  TranslationCartesianOffset=[1.3358203432289883e-12 0 -1.0913936421275139e-11]  TranslationROffset=0  TranslationROffsetUnits=m  TranslationZOffset=0  TranslationZOffsetUnits=m  TranslationThetaOffset=0  TranslationThetaOffsetUnits=deg  RotationMethod=None  RotationAngleUnits=rad  RotationStandardAxis=+X  RotationAngle=pi/2  RotationArbitraryAxis=[0 0 0]  FollAlignAxisA=+X  BaseAlignAxisA=+Y  FollAlignAxisB=+Y  BaseAlignAxisB=+Z  BlockFunction=simmechanics.library.frames_transforms.rigid_transform
  F : PMIOPort  Port=1  Side=Right
  B : PMIOPort  Port=2  Side=Left
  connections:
  Transform/LConn1 -- Transform1/LConn1 -- ReferenceFrame/RConn1 -- Solid/RConn1
  Transform/RConn1 -- B/RConn1
  Transform1/RConn1 -- F/RConn1

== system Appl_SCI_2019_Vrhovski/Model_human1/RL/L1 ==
  Mux : Mux  Inputs=3
  Pos X Converter : nesl_utility/PS-Simulink Converter  PhysicalDomain=network_engine_domain  SubClassName=ps_output  LeftPortType=input  RightPortType=output  PseudoPeriodic=off  Frequencies=[]  Unit=mm  AffineConversion=off
  Pos Y Converter : nesl_utility/PS-Simulink Converter  PhysicalDomain=network_engine_domain  SubClassName=ps_output  LeftPortType=input  RightPortType=output  PseudoPeriodic=off  Frequencies=[]  Unit=mm  AffineConversion=off
  Pos Z Converter2 : nesl_utility/PS-Simulink Converter  PhysicalDomain=network_engine_domain  SubClassName=ps_output  LeftPortType=input  RightPortType=output  PseudoPeriodic=off  Frequencies=[]  Unit=mm  AffineConversion=off
  Transform Sensor : sm_lib/Frames and Transforms/Transform Sensor  MeasurementFrame=World  SenseAngle=off  SenseAxis=off  SenseAngle1=off  SenseAngle2=off  SenseAngle3=off  SenseQ=off  SenseR=off  SenseOmegaX=off  SenseOmegaY=off  SenseOmegaZ=off  SenseOmega1=off  SenseOmega2=off  SenseOmega3=off  SenseQDot=off  SenseRDot=off  SenseAlphaX=off  SenseAlphaY=off  SenseAlphaZ=off  SenseAlpha1=off  SenseAlpha2=off  SenseAlpha3=off  SenseQDDot=off  SenseRDDot=off  SenseX=on  SenseY=on  SenseZ=on  SenseRad=on  SenseAzim=off  SenseDist=off  SenseInc=off  SenseXDot=off  SenseYDot=off  SenseZDot=off  SenseRadDot=off  SenseAzimDot=off  SenseDistDot=off  SenseIncDot=off  SenseXDDot=off  SenseYDDot=off  SenseZDDot=off  SenseRadDDot=off  SenseAzimDDot=off  SenseDistDDot=off  SenseIncDDot=off  BlockFunction=simmechanics.library.frames_transforms.transform_sensor
  base_coord_sys : PMIOPort  Port=1  Side=Left
  marker : PMIOPort  Port=2  Side=Left
  xyz : Outport
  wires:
  Mux/1 -> xyz/1
  Pos Y Converter/1 -> Mux/2
  Pos X Converter/1 -> Mux/1
  Pos Z Converter2/1 -> Mux/3
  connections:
  Transform Sensor/RConn3 -- Pos Y Converter/LConn1
  Pos X Converter/LConn1 -- Transform Sensor/RConn2
  Pos Z Converter2/LConn1 -- Transform Sensor/RConn4
  marker/RConn1 -- Transform Sensor/RConn1
  base_coord_sys/RConn1 -- Transform Sensor/LConn1

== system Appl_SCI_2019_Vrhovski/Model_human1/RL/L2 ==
  Mux : Mux  Inputs=3
  Pos X Converter : nesl_utility/PS-Simulink Converter  PhysicalDomain=network_engine_domain  SubClassName=ps_output  LeftPortType=input  RightPortType=output  PseudoPeriodic=off  Frequencies=[]  Unit=mm  AffineConversion=off
  Pos Y Converter : nesl_utility/PS-Simulink Converter  PhysicalDomain=network_engine_domain  SubClassName=ps_output  LeftPortType=input  RightPortType=output  PseudoPeriodic=off  Frequencies=[]  Unit=mm  AffineConversion=off
  Pos Z Converter2 : nesl_utility/PS-Simulink Converter  PhysicalDomain=network_engine_domain  SubClassName=ps_output  LeftPortType=input  RightPortType=output  PseudoPeriodic=off  Frequencies=[]  Unit=mm  AffineConversion=off
  Transform Sensor : sm_lib/Frames and Transforms/Transform Sensor  MeasurementFrame=World  SenseAngle=off  SenseAxis=off  SenseAngle1=off  SenseAngle2=off  SenseAngle3=off  SenseQ=off  SenseR=off  SenseOmegaX=off  SenseOmegaY=off  SenseOmegaZ=off  SenseOmega1=off  SenseOmega2=off  SenseOmega3=off  SenseQDot=off  SenseRDot=off  SenseAlphaX=off  SenseAlphaY=off  SenseAlphaZ=off  SenseAlpha1=off  SenseAlpha2=off  SenseAlpha3=off  SenseQDDot=off  SenseRDDot=off  SenseX=on  SenseY=on  SenseZ=on  SenseRad=on  SenseAzim=off  SenseDist=off  SenseInc=off  SenseXDot=off  SenseYDot=off  SenseZDot=off  SenseRadDot=off  SenseAzimDot=off  SenseDistDot=off  SenseIncDot=off  SenseXDDot=off  SenseYDDot=off  SenseZDDot=off  SenseRadDDot=off  SenseAzimDDot=off  SenseDistDDot=off  SenseIncDDot=off  BlockFunction=simmechanics.library.frames_transforms.transform_sensor
  base_coord_sys : PMIOPort  Port=1  Side=Left
  marker : PMIOPort  Port=2  Side=Left
  xyz : Outport
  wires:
  Pos Z Converter2/1 -> Mux/3
  Pos X Converter/1 -> Mux/1
  Pos Y Converter/1 -> Mux/2
  Mux/1 -> xyz/1
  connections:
  base_coord_sys/RConn1 -- Transform Sensor/LConn1
  marker/RConn1 -- Transform Sensor/RConn1
  Pos Z Converter2/LConn1 -- Transform Sensor/RConn4
  Pos X Converter/LConn1 -- Transform Sensor/RConn2
  Transform Sensor/RConn3 -- Pos Y Converter/LConn1

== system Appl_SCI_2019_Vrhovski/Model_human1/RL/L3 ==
  Mux : Mux  Inputs=3
  Pos X Converter : nesl_utility/PS-Simulink Converter  PhysicalDomain=network_engine_domain  SubClassName=ps_output  LeftPortType=input  RightPortType=output  PseudoPeriodic=off  Frequencies=[]  Unit=mm  AffineConversion=off
  Pos Y Converter : nesl_utility/PS-Simulink Converter  PhysicalDomain=network_engine_domain  SubClassName=ps_output  LeftPortType=input  RightPortType=output  PseudoPeriodic=off  Frequencies=[]  Unit=mm  AffineConversion=off
  Pos Z Converter2 : nesl_utility/PS-Simulink Converter  PhysicalDomain=network_engine_domain  SubClassName=ps_output  LeftPortType=input  RightPortType=output  PseudoPeriodic=off  Frequencies=[]  Unit=mm  AffineConversion=off
  Transform Sensor : sm_lib/Frames and Transforms/Transform Sensor  MeasurementFrame=World  SenseAngle=off  SenseAxis=off  SenseAngle1=off  SenseAngle2=off  SenseAngle3=off  SenseQ=off  SenseR=off  SenseOmegaX=off  SenseOmegaY=off  SenseOmegaZ=off  SenseOmega1=off  SenseOmega2=off  SenseOmega3=off  SenseQDot=off  SenseRDot=off  SenseAlphaX=off  SenseAlphaY=off  SenseAlphaZ=off  SenseAlpha1=off  SenseAlpha2=off  SenseAlpha3=off  SenseQDDot=off  SenseRDDot=off  SenseX=on  SenseY=on  SenseZ=on  SenseRad=on  SenseAzim=off  SenseDist=off  SenseInc=off  SenseXDot=off  SenseYDot=off  SenseZDot=off  SenseRadDot=off  SenseAzimDot=off  SenseDistDot=off  SenseIncDot=off  SenseXDDot=off  SenseYDDot=off  SenseZDDot=off  SenseRadDDot=off  SenseAzimDDot=off  SenseDistDDot=off  SenseIncDDot=off  BlockFunction=simmechanics.library.frames_transforms.transform_sensor
  base_coord_sys : PMIOPort  Port=1  Side=Left
  marker : PMIOPort  Port=2  Side=Left
  xyz : Outport
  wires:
  Mux/1 -> xyz/1
  Pos Y Converter/1 -> Mux/2
  Pos X Converter/1 -> Mux/1
  Pos Z Converter2/1 -> Mux/3
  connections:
  Transform Sensor/RConn3 -- Pos Y Converter/LConn1
  Pos X Converter/LConn1 -- Transform Sensor/RConn2
  Pos Z Converter2/LConn1 -- Transform Sensor/RConn4
  marker/RConn1 -- Transform Sensor/RConn1
  base_coord_sys/RConn1 -- Transform Sensor/LConn1

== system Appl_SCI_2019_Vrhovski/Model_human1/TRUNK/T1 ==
  Mux : Mux  Inputs=3
  Pos X Converter : nesl_utility/PS-Simulink Converter  PhysicalDomain=network_engine_domain  SubClassName=ps_output  LeftPortType=input  RightPortType=output  PseudoPeriodic=off  Frequencies=[]  Unit=mm  AffineConversion=off
  Pos Y Converter : nesl_utility/PS-Simulink Converter  PhysicalDomain=network_engine_domain  SubClassName=ps_output  LeftPortType=input  RightPortType=output  PseudoPeriodic=off  Frequencies=[]  Unit=mm  AffineConversion=off
  Pos Z Converter2 : nesl_utility/PS-Simulink Converter  PhysicalDomain=network_engine_domain  SubClassName=ps_output  LeftPortType=input  RightPortType=output  PseudoPeriodic=off  Frequencies=[]  Unit=mm  AffineConversion=off
  Transform Sensor : sm_lib/Frames and Transforms/Transform Sensor  MeasurementFrame=World  SenseAngle=off  SenseAxis=off  SenseAngle1=off  SenseAngle2=off  SenseAngle3=off  SenseQ=off  SenseR=off  SenseOmegaX=off  SenseOmegaY=off  SenseOmegaZ=off  SenseOmega1=off  SenseOmega2=off  SenseOmega3=off  SenseQDot=off  SenseRDot=off  SenseAlphaX=off  SenseAlphaY=off  SenseAlphaZ=off  SenseAlpha1=off  SenseAlpha2=off  SenseAlpha3=off  SenseQDDot=off  SenseRDDot=off  SenseX=on  SenseY=on  SenseZ=on  SenseRad=on  SenseAzim=off  SenseDist=off  SenseInc=off  SenseXDot=off  SenseYDot=off  SenseZDot=off  SenseRadDot=off  SenseAzimDot=off  SenseDistDot=off  SenseIncDot=off  SenseXDDot=off  SenseYDDot=off  SenseZDDot=off  SenseRadDDot=off  SenseAzimDDot=off  SenseDistDDot=off  SenseIncDDot=off  BlockFunction=simmechanics.library.frames_transforms.transform_sensor
  base_coord_sys : PMIOPort  Port=1  Side=Left
  marker : PMIOPort  Port=2  Side=Left
  xyz : Outport
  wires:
  Pos Z Converter2/1 -> Mux/3
  Pos X Converter/1 -> Mux/1
  Pos Y Converter/1 -> Mux/2
  Mux/1 -> xyz/1
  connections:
  base_coord_sys/RConn1 -- Transform Sensor/LConn1
  marker/RConn1 -- Transform Sensor/RConn1
  Pos Z Converter2/LConn1 -- Transform Sensor/RConn4
  Pos X Converter/LConn1 -- Transform Sensor/RConn2
  Transform Sensor/RConn3 -- Pos Y Converter/LConn1
